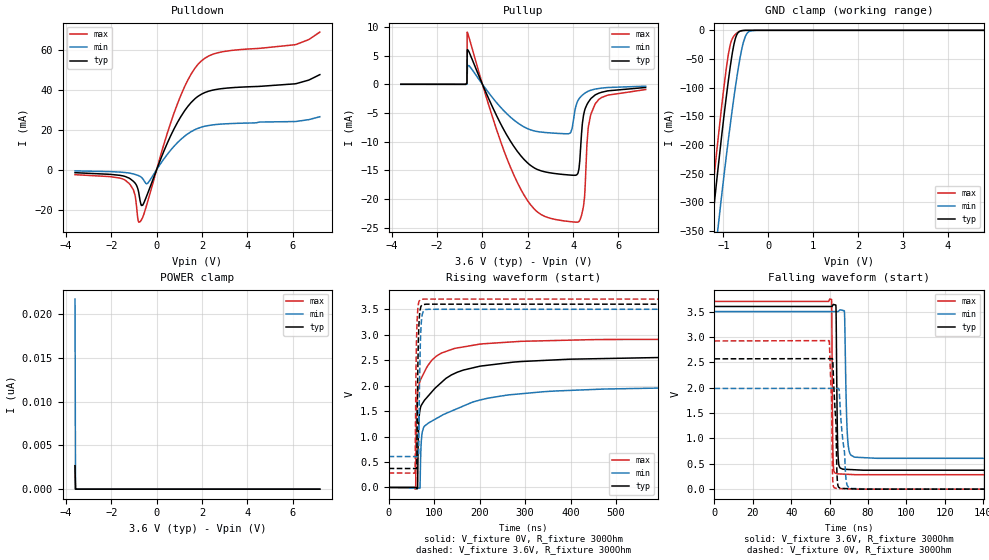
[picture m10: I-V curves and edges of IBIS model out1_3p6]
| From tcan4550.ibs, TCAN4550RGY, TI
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|   out1 Model
[Model]   out1_3p6
Model_type   3-state
Polarity   Non-Inverting
Vmeas = 1.8
Vref = 0
Cref = 2pF
Rref = 100000
|   typ   min   max
C_comp   5.830pF   5.542pF   5.965pF
|  Where Nom  PVT is Nominal Process, 3.6V, 27C
|   Fast PVT is Strong Process,  3.7, -40C
|   Slow PVT is Weak Process,   3.5V, 150C
[Voltage Range]   3.6   3.5   3.7
|Junction Temperature
[Temperature Range]   27   150   -40
[Pullup Reference]   3.6   3.5   3.7
[Pulldown Reference]   0   0   0
[Power Clamp Reference]   3.6   3.5   3.7
[GND Clamp Reference]   0   0   0
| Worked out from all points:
|   slope of the pulldown table from 0 to 0.54 V, typ, clamps not added: 35.9 ohm
|   slope of the pullup table from 0 to 0.54 V, typ, clamps not added: 113 ohm
|   GND clamp passes 1 mA (typ) near -0.61 V on its own axis
|   falling waveform, V_fixture 3.6V, R_fixture 300Ohm: 20-80 % time 583ps typ, 1.04ns min, 402ps max; typ from 3.6 V to 0.374 V
|   rising waveform, V_fixture 0V, R_fixture 300Ohm: 20-80 % time 50.7ns typ, 91.4ns min, 22.5ns max; typ from 0 V to 2.57 V
|   rising waveform, V_fixture 3.6V, R_fixture 300Ohm: 20-80 % time 3.07ns typ, 3.38ns min, 2.92ns max; typ from 0.374 V to 3.6 V
|   falling waveform, V_fixture 0V, R_fixture 300Ohm: 20-80 % time 1.52ns typ, 2.63ns min, 998ps max; typ from 2.57 V to 0 V
[Pulldown]
|   Voltage   I(typ)   I(min)   I(max)
-3.6V     -1.499mA   -600.9uA   -2.506mA
-1.397V   -3.362mA   -1.414mA   -5.162mA
-1.019V   -5.895mA   -2.161mA   -10.27mA
-813.6mV  -10.25mA   -2.918mA   -25.51mA
-738mV    -14.99mA   -3.313mA   -26.17mA
-619.2mV  -17.85mA   -4.43mA    -24.02mA
-403.2mV  -12.13mA   -6.869mA   -16.3mA
774mV     20.59mA    11.82mA    28.56mA
1.832V    36.83mA    20.77mA    52.89mA
2.61V     40.19mA    22.63mA    58.33mA
6.098V    43.03mA    24.13mA    62.63mA
7.2V      47.64mA    26.54mA    68.98mA
[GND Clamp]
|   Voltage   I(typ)   I(min)   I(max)
-3.6V     -2.295A    -2.312A    -2.301A
-1.31V    -383.7mA   -482.6mA   -335.3mA
-1.224V   -317.5mA   -418.8mA   -267.6mA
-1.138V   -253.5mA   -356.4mA   -202.7mA
-1.051V   -192.3mA   -296.1mA   -140.9mA
-889.2mV  -87.18mA   -190.1mA   -41.57mA
-835.2mV  -56.62mA   -157.2mA   -21.58mA
-759.6mV  -22.39mA   -113.5mA   -9.313mA
-630mV    -1.471mA   -48.31mA   -1.464mA
-500.4mV  -60.15uA   -8.767mA   -60.67uA
-284.4mV  -1.206uA   -50.38uA   0A
7.2V      0A         0A         0A
[Pullup]
|   Voltage   I(typ)   I(min)   I(max)
-3.6V     14.39uA    11.62uA    19.39uA
-738mV    8.59uA     6.849uA    11.7uA
-684mV    196.9uA    14.53uA    338.5uA
-673.2mV  5.975mA    1.506mA    9.131mA
774mV     -6.669mA   -3.884mA   -9.656mA
1.832V    -13.1mA    -7.426mA   -19.31mA
3.798V    -15.81mA   -8.624mA   -23.94mA
4.154V    -15.8mA    -3.371mA   -24.07mA
4.5V      -4.646mA   -1.583mA   -19.82mA
4.662V    -3.157mA   -1.201mA   -7.749mA
4.975V    -1.835mA   -818.6uA   -3.397mA
7.2V      -539.8uA   -314.8uA   -903.9uA
[POWER Clamp]
|   Voltage   I(typ)   I(min)   I(max)
-3.6V     2.678nA    21.76nA    2.692nA
-3.578V   0A         0A         0A
-3.568V   0A         0A         0A
7.2V      0A         0A         0A
[Ramp]
R_load = 300
|   typ   min   max
dV/dt_r   1.54093/4.96808e-08   1.19092/8.75599e-08   1.75253/2.2474e-08
dV/dt_f   1.93586/5.81364e-10   1.73529/1.03032e-09   2.04894/4.01469e-10
[Falling Waveform]
V_fixture = 3.6V
V_fixture_min = 3.5V
V_fixture_max = 3.7V
R_fixture = 300Ohm
C_fixture = 0F
|   Time   V(typ)   V(min)   V(max)
0s        3.6V       3.5V       3.7V
61.04ns   3.6V       3.5V       3.738V
61.62ns   3.622V     3.5V       1.014V
62.16ns   3.639V     3.5V       374.8mV
63.34ns   3.588V     3.5V       311.9mV
64.82ns   481.6mV    3.512V     300.7mV
67.77ns   392.1mV    3.476V     295.5mV
69.75ns   388.4mV    847.1mV    291.9mV
73.4ns    381.6mV    629.4mV    285.5mV
25us      373.6mV    607.8mV    285.1mV
[Rising Waveform]
V_fixture = 0V
V_fixture_min = 0V
V_fixture_max = 0V
R_fixture = 300Ohm
C_fixture = 0F
|   Time   V(typ)   V(min)   V(max)
0s        -111.5nV   759.6nV    7.16nV
59.5ns    715.9uV    -10.49mV   -23.99mV
61.38ns   738.6uV    -10.83mV   1.438V
63.76ns   -16.9mV    -11.25mV   1.876V
64.81ns   754.6mV    -11.43mV   1.948V
68.95ns   1.52V      -12.16mV   2.079V
74.02ns   1.645V     1.092V     2.182V
104.7ns   1.971V     1.353V     2.577V
442.4ns   2.526V     1.922V     2.902V
25us      2.568V     1.985V     2.921V
[Rising Waveform]
V_fixture = 3.6V
V_fixture_min = 3.5V
V_fixture_max = 3.7V
R_fixture = 300Ohm
C_fixture = 0F
|   Time   V(typ)   V(min)   V(max)
0s        373.6mV    607.8mV    285.1mV
58.22ns   371.4mV    606.5mV    281.2mV
60.08ns   371.3mV    606.4mV    2.193V
61.95ns   371.3mV    606.4mV    3.08V
64.46ns   2.463V     606.3mV    3.526V
66.36ns   3.136V     757mV      3.637V
67.89ns   3.381V     2.006V     3.668V
70.01ns   3.516V     2.882V     3.689V
76.4ns    3.592V     3.462V     3.699V
25us      3.6V       3.5V       3.7V
[Falling Waveform]
|Gnd
V_fixture = 0V
V_fixture_min = 0V
V_fixture_max = 0V
R_fixture = 300Ohm
C_fixture = 0F
|   Time   V(typ)   V(min)   V(max)
0s        2.568V     1.985V     2.921V
59.75ns   2.572V     1.986V     2.927V
61.08ns   2.572V     1.986V     1.762V
61.47ns   2.572V     1.986V     420.8mV
61.9ns    2.32V      1.986V     70.18mV
63.33ns   1.311V     1.986V     17.64mV
64.34ns   76.51mV    1.986V     12.49mV
68.76ns   11.41mV    139.6mV    6.555mV
73.4ns    4.59mV     11.62mV    327.7uV
25us      -398.1nV   749.8nV    7.156nV
